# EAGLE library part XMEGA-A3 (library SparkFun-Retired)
Atmel's 8/16-bit AVR XMEGA A3 Microcontroller - ATxmega256A3, etc. Retired: IC-09806 - ATXMEGA256A3 Retired: IC-09429 - ATXMEGA128A1
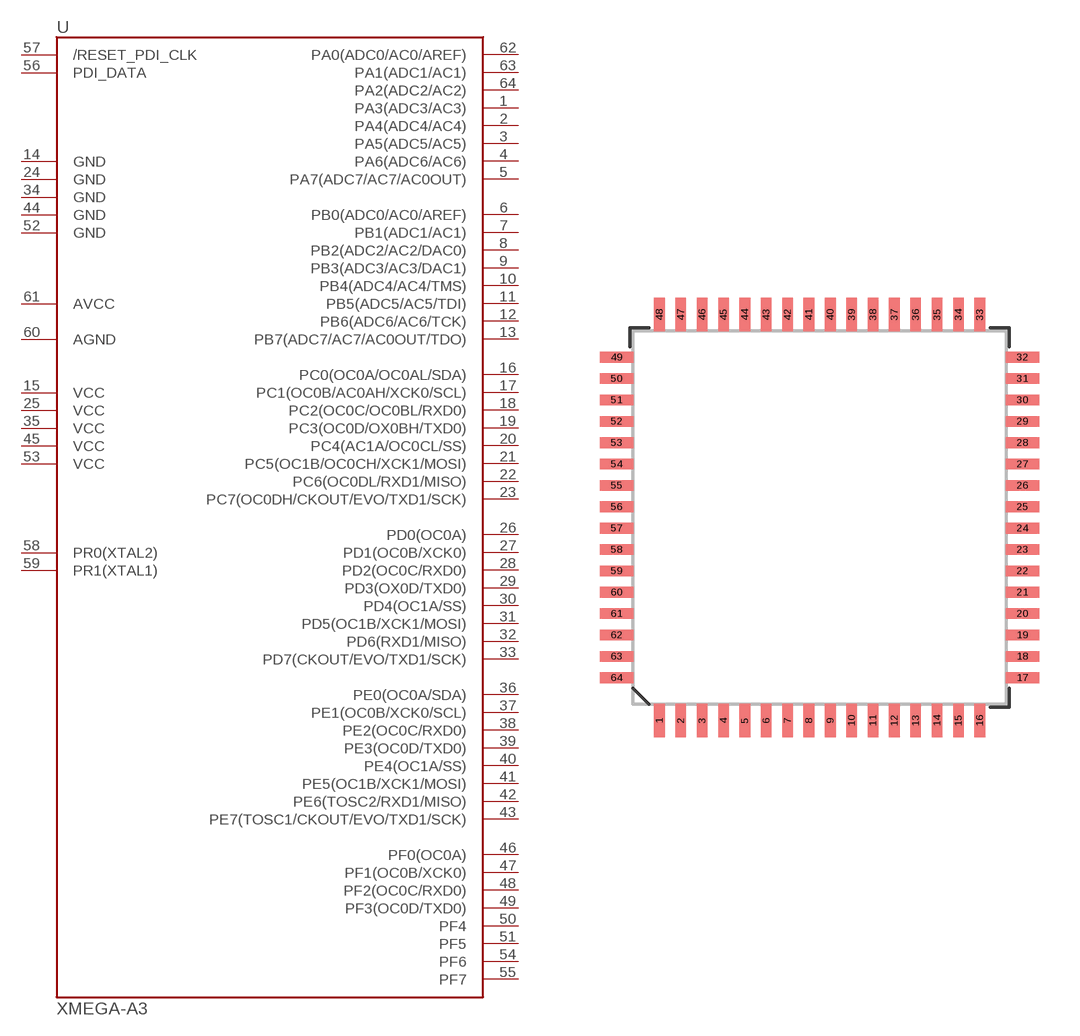
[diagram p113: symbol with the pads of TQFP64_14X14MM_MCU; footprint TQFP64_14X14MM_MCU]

Designator prefix -

## XMEGA-A3-AU  [TQFP64_14X14MM_MCU]
1  PA3(ADC3/AC3)
2  PA4(ADC4/AC4)
3  PA5(ADC5/AC5)
4  PA6(ADC6/AC6)
5  PA7(ADC7/AC7/AC0OUT)
6  PB0(ADC0/AC0/AREF)
7  PB1(ADC1/AC1)
8  PB2(ADC2/AC2/DAC0)
9  PB3(ADC3/AC3/DAC1)
10  PB4(ADC4/AC4/TMS)
11  PB5(ADC5/AC5/TDI)
12  PB6(ADC6/AC6/TCK)
13  PB7(ADC7/AC7/AC0OUT/TDO)
14  GND1
15  VCC1
16  PC0(OC0A/OC0AL/SDA)
17  PC1(OC0B/AC0AH/XCK0/SCL)
18  PC2(OC0C/OC0BL/RXD0)
19  PC3(OC0D/OX0BH/TXD0)
20  PC4(AC1A/OC0CL/SS)
21  PC5(OC1B/OC0CH/XCK1/MOSI)
22  PC6(OC0DL/RXD1/MISO)
23  PC7(OC0DH/CKOUT/EVO/TXD1/SCK)
24  GND2
25  VCC2
26  PD0(OC0A)
27  PD1(OC0B/XCK0)
28  PD2(OC0C/RXD0)
29  PD3(OX0D/TXD0)
30  PD4(OC1A/SS)
31  PD5(OC1B/XCK1/MOSI)
32  PD6(RXD1/MISO)
33  PD7(CKOUT/EVO/TXD1/SCK)
34  GND3
35  VCC3
36  PE0(OC0A/SDA)
37  PE1(OC0B/XCK0/SCL)
38  PE2(OC0C/RXD0)
39  PE3(OC0D/TXD0)
40  PE4(OC1A/SS)
41  PE5(OC1B/XCK1/MOSI)
42  PE6(TOSC2/RXD1/MISO)
43  PE7(TOSC1/CKOUT/EVO/TXD1/SCK)
44  GND4
45  VCC4
46  PF0(OC0A)
47  PF1(OC0B/XCK0)
48  PF2(OC0C/RXD0)
49  PF3(OC0D/TXD0)
50  PF4
51  PF5
52  GND5
53  VCC5
54  PF6
55  PF7
56  PDI_DATA
57  /RESET_PDI_CLK
58  PR0(XTAL2)
59  PR1(XTAL1)
60  AGND
61  AVCC
62  PA0(ADC0/AC0/AREF)
63  PA1(ADC1/AC1)
64  PA2(ADC2/AC2)

## Footprint TQFP64_14X14MM_MCU (pad centres in mm)
64-Lead TQFP Plastic Thin Quad Flatpack - 14x14x1mm Body
smd 0.4 x 1.27: 1 -6,-7.6; 2 -5.2,-7.6; 3 -4.4,-7.6; 4 -3.6,-7.6; 5 -2.8,-7.6; 6 -2,-7.6; 7 -1.2,-7.6; 8 -0.4,-7.6; 9 0.4,-7.6; 10 1.2,-7.6; 11 2,-7.6; 12 2.8,-7.6; 13 3.6,-7.6; 14 4.4,-7.6; 15 5.2,-7.6; 16 6,-7.6; 33 6,7.6; 34 5.2,7.6; 35 4.4,7.6; 36 3.6,7.6; 37 2.8,7.6; 38 2,7.6; 39 1.2,7.6; 40 0.4,7.6; 41 -0.4,7.6; 42 -1.2,7.6; 43 -2,7.6; 44 -2.8,7.6; 45 -3.6,7.6; 46 -4.4,7.6; 47 -5.2,7.6; 48 -6,7.6
smd 1.27 x 0.4: 17 7.6,-6; 18 7.6,-5.2; 19 7.6,-4.4; 20 7.6,-3.6; 21 7.6,-2.8; 22 7.6,-2; 23 7.6,-1.2; 24 7.6,-0.4; 25 7.6,0.4; 26 7.6,1.2; 27 7.6,2; 28 7.6,2.8; 29 7.6,3.6; 30 7.6,4.4; 31 7.6,5.2; 32 7.6,6; 49 -7.6,6; 50 -7.6,5.2; 51 -7.6,4.4; 52 -7.6,3.6; 53 -7.6,2.8; 54 -7.6,2; 55 -7.6,1.2; 56 -7.6,0.4; 57 -7.6,-0.4; 58 -7.6,-1.2; 59 -7.6,-2; 60 -7.6,-2.8; 61 -7.6,-3.6; 62 -7.6,-4.4; 63 -7.6,-5.2; 64 -7.6,-6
